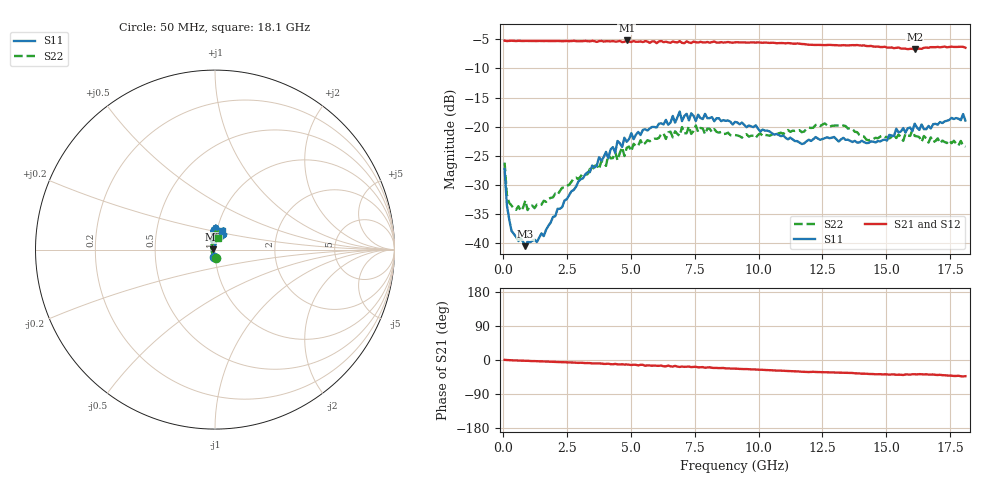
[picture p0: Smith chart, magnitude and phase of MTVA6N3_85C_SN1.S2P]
! Network Analyzer HP8720D.06.14 Serial No. US36140669
!  5 Jul 2005  10:29:57
! Frequency  S11  S21  S12  S22
# HZ  S  DB R 50
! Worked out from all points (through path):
!   201 points, 50 MHz to 18.1 GHz, reference 50 ohm
!   highest |S21| = -5.21 dB at 4.833 GHz (marker M1); lowest = -6.7 dB at 16.11 GHz (marker M2)
!   group delay of S21, straight-line fit = 6.75 ps
!   lowest |S11| = -40.5 dB at 862.2 MHz (marker M3), VSWR 1.02, Z = 49.1 + j0.238 ohm
!   |S11| at or under -10 dB: start of sweep to end of sweep
!   |S22| runs from -34.4 to -19.4 dB; largest |S21 - S12| = 0.019
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5e7  -27.21 -95.0  -5.24 0.3  -5.26 0.6  -26.15 -86.6
1.4025e8  -33.49 -111.7  -5.31 -0.1  -5.29 -0.1  -31.71 -128.2
3.2075e8  -37.84 -138.4  -5.26 -0.6  -5.28 -0.6  -33.50 -154.1
6.8175e8  -39.13 -177.4  -5.29 -1.6  -5.31 -1.6  -34.43 -177.1
8.6225e8  -40.47 165.2  -5.29 -2.0  -5.30 -2.0  -32.65 177.2
1.22325e9  -39.36 148.0  -5.31 -2.9  -5.32 -3.0  -33.95 160.8
1.58425e9  -38.74 121.3  -5.31 -3.9  -5.31 -3.9  -32.69 148.6
3.1185e9  -28.85 88.1  -5.32 -7.6  -5.34 -7.8  -28.00 121.7
3.75025e9  -25.22 83.9  -5.32 -9.2  -5.36 -8.8  -27.28 111.8
4.382e9  -24.45 81.4  -5.40 -10.3  -5.36 -11.3  -24.33 108.1
4.47225e9  -22.43 77.8  -5.38 -11.4  -5.33 -10.7  -25.75 109.9
4.83325e9  -22.58 86.9  -5.21 -11.8  -5.31 -12.6  -23.58 96.3
6.09675e9  -19.47 83.3  -5.38 -15.4  -5.32 -15.3  -21.90 92.4
6.7285e9  -19.29 89.5  -5.50 -15.5  -5.64 -16.5  -20.78 87.0
6.909e9  -17.39 88.1  -5.32 -18.3  -5.45 -17.4  -21.57 85.0
6.99925e9  -19.03 87.2  -5.61 -17.2  -5.66 -18.6  -20.05 87.2
7.54075e9  -19.02 85.7  -5.51 -17.8  -5.38 -19.6  -19.78 90.8
9.075e9  -19.17 98.3  -5.53 -22.8  -5.51 -22.9  -21.42 80.1
1.21435e10  -22.13 90.6  -5.96 -31.2  -5.92 -31.5  -20.15 76.8
1.512175e10  -21.39 56.2  -6.44 -38.6  -6.33 -38.3  -22.00 81.5
1.61145e10  -19.47 53.2  -6.74 -37.6  -6.54 -38.2  -21.57 72.3
1.81e10  -18.94 69.7  -6.45 -42.7  -6.51 -43.8  -23.42 77.8
